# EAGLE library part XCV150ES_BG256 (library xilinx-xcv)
xcv150es_bg256 edit this description Auto generated by make-symbol-device-package-bsdl.ulp Rev. 26 Source: xcv150es_bg256.bsd
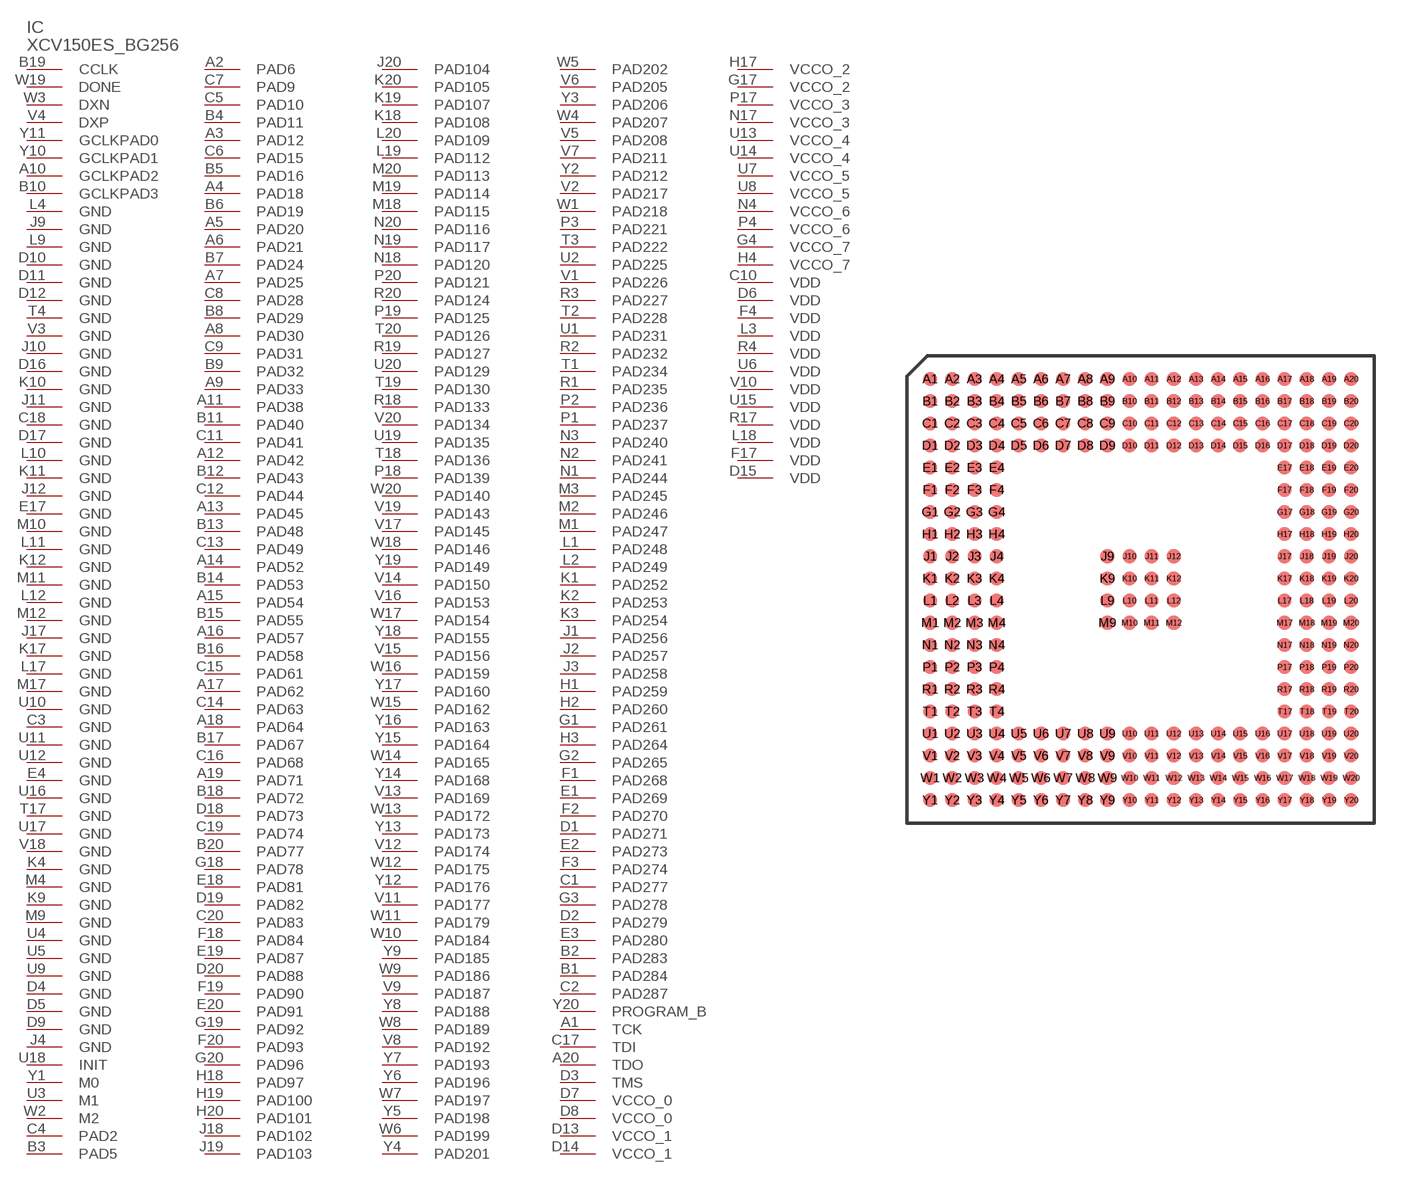
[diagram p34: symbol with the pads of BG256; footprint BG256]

Designator prefix IC

## XCV150ES_BG256 (OC_FARNELL: unknown; OC_NEWARK: unknown)  [BG256]
A1  TCK  in
A2  PAD6
A3  PAD12
A4  PAD18
A5  PAD20
A6  PAD21
A7  PAD25
A8  PAD30
A9  PAD33
A10  GCLKPAD2  in
A11  PAD38
A12  PAD42
A13  PAD45
A14  PAD52
A15  PAD54
A16  PAD57
A17  PAD62
A18  PAD64
A19  PAD71
A20  TDO  out
B1  PAD284
B2  PAD283
B3  PAD5
B4  PAD11
B5  PAD16
B6  PAD19
B7  PAD24
B8  PAD29
B9  PAD32
B10  GCLKPAD3  in
B11  PAD40
B12  PAD43
B13  PAD48
B14  PAD53
B15  PAD55
B16  PAD58
B17  PAD67
B18  PAD72
B19  CCLK
B20  PAD77
C1  PAD277
C2  PAD287
C3  GND  pwr
C4  PAD2
C5  PAD10
C6  PAD15
C7  PAD9
C8  PAD28
C9  PAD31
C10  VDD  pwr
C11  PAD41
C12  PAD44
C13  PAD49
C14  PAD63
C15  PAD61
C16  PAD68
C17  TDI  in
C18  GND  pwr
C19  PAD74
C20  PAD83
D1  PAD271
D2  PAD279
D3  TMS  in
D4  GND  pwr
D5  GND  pwr
D6  VDD  pwr
D7  VCCO_0  pwr
D8  VCCO_0  pwr
D9  GND  pwr
D10  GND  pwr
D11  GND  pwr
D12  GND  pwr
D13  VCCO_1  pwr
D14  VCCO_1  pwr
D15  VDD  pwr
D16  GND  pwr
D17  GND  pwr
D18  PAD73
D19  PAD82
D20  PAD88
E1  PAD269
E2  PAD273
E3  PAD280
E4  GND  pwr
E17  GND  pwr
E18  PAD81
E19  PAD87
E20  PAD91
F1  PAD268
F2  PAD270
F3  PAD274
F4  VDD  pwr
F17  VDD  pwr
F18  PAD84
F19  PAD90
F20  PAD93
G1  PAD261
G2  PAD265
G3  PAD278
G4  VCCO_7  pwr
G17  VCCO_2  pwr
G18  PAD78
G19  PAD92
G20  PAD96
H1  PAD259
H2  PAD260
H3  PAD264
H4  VCCO_7  pwr
H17  VCCO_2  pwr
H18  PAD97
H19  PAD100
H20  PAD101
J1  PAD256
J2  PAD257
J3  PAD258
J4  GND  pwr
J9  GND  pwr
J10  GND  pwr
J11  GND  pwr
J12  GND  pwr
J17  GND  pwr
J18  PAD102
J19  PAD103
J20  PAD104
K1  PAD252
K2  PAD253
K3  PAD254
K4  GND  pwr
K9  GND  pwr
K10  GND  pwr
K11  GND  pwr
K12  GND  pwr
K17  GND  pwr
K18  PAD108
K19  PAD107
K20  PAD105
L1  PAD248
L2  PAD249
L3  VDD  pwr
L4  GND  pwr
L9  GND  pwr
L10  GND  pwr
L11  GND  pwr
L12  GND  pwr
L17  GND  pwr
L18  VDD  pwr
L19  PAD112
L20  PAD109
M1  PAD247
M2  PAD246
M3  PAD245
M4  GND  pwr
M9  GND  pwr
M10  GND  pwr
M11  GND  pwr
M12  GND  pwr
M17  GND  pwr
M18  PAD115
M19  PAD114
M20  PAD113
N1  PAD244
N2  PAD241
N3  PAD240
N4  VCCO_6  pwr
N17  VCCO_3  pwr
N18  PAD120
N19  PAD117
N20  PAD116
P1  PAD237
P2  PAD236
P3  PAD221
P4  VCCO_6  pwr
P17  VCCO_3  pwr
P18  PAD139
P19  PAD125
P20  PAD121
R1  PAD235
R2  PAD232
R3  PAD227
R4  VDD  pwr
R17  VDD  pwr
R18  PAD133
R19  PAD127
R20  PAD124
T1  PAD234
T2  PAD228
T3  PAD222
T4  GND  pwr
T17  GND  pwr
T18  PAD136
T19  PAD130
T20  PAD126
U1  PAD231
U2  PAD225
U3  M1  in
U4  GND  pwr
U5  GND  pwr
U6  VDD  pwr
U7  VCCO_5  pwr
U8  VCCO_5  pwr
U9  GND  pwr
U10  GND  pwr
U11  GND  pwr
U12  GND  pwr
U13  VCCO_4  pwr
U14  VCCO_4  pwr
U15  VDD  pwr
U16  GND  pwr
U17  GND  pwr
U18  INIT
U19  PAD135
U20  PAD129
V1  PAD226
V2  PAD217
V3  GND  pwr
V4  DXP  pas
V5  PAD208
V6  PAD205
V7  PAD211
V8  PAD192
V9  PAD187
V10  VDD  pwr
V11  PAD177
V12  PAD174
V13  PAD169
V14  PAD150
V15  PAD156
V16  PAD153
V17  PAD145
V18  GND  pwr
V19  PAD143
V20  PAD134
W1  PAD218
W2  M2  in
W3  DXN  pas
W4  PAD207
W5  PAD202
W6  PAD199
W7  PAD197
W8  PAD189
W9  PAD186
W10  PAD184
W11  PAD179
W12  PAD175
W13  PAD172
W14  PAD165
W15  PAD162
W16  PAD159
W17  PAD154
W18  PAD146
W19  DONE
W20  PAD140
Y1  M0  in
Y2  PAD212
Y3  PAD206
Y4  PAD201
Y5  PAD198
Y6  PAD196
Y7  PAD193
Y8  PAD188
Y9  PAD185
Y10  GCLKPAD1  in
Y11  GCLKPAD0  in
Y12  PAD176
Y13  PAD173
Y14  PAD168
Y15  PAD164
Y16  PAD163
Y17  PAD160
Y18  PAD155
Y19  PAD149
Y20  PROGRAM_B  in

## Footprint BG256 (pad centres in mm)
xcv100_bg256_1532 edit this description Auto generated by make-symbol-device-package-bsdl.ulp Rev. 25 Source: xcv100_bg256_1532.bsd
smd 0.8 x 0.8: A1 -12.065,12.065; A2 -10.795,12.065; A3 -9.525,12.065; A4 -8.255,12.065; A5 -6.985,12.065; A6 -5.715,12.065; A7 -4.445,12.065; A8 -3.175,12.065; A9 -1.905,12.065; A10 -0.635,12.065; A11 0.635,12.065; A12 1.905,12.065; A13 3.175,12.065; A14 4.445,12.065; A15 5.715,12.065; A16 6.985,12.065; A17 8.255,12.065; A18 9.525,12.065; A19 10.795,12.065; A20 12.065,12.065; B1 -12.065,10.795; B2 -10.795,10.795; B3 -9.525,10.795; B4 -8.255,10.795; B5 -6.985,10.795; B6 -5.715,10.795; B7 -4.445,10.795; B8 -3.175,10.795; B9 -1.905,10.795; B10 -0.635,10.795; B11 0.635,10.795; B12 1.905,10.795; B13 3.175,10.795; B14 4.445,10.795; B15 5.715,10.795; B16 6.985,10.795; B17 8.255,10.795; B18 9.525,10.795; B19 10.795,10.795; B20 12.065,10.795; C1 -12.065,9.525; C2 -10.795,9.525; C3 -9.525,9.525; C4 -8.255,9.525; C5 -6.985,9.525; C6 -5.715,9.525; C7 -4.445,9.525; C8 -3.175,9.525; C9 -1.905,9.525; C10 -0.635,9.525; C11 0.635,9.525; C12 1.905,9.525; C13 3.175,9.525; C14 4.445,9.525; C15 5.715,9.525; C16 6.985,9.525; C17 8.255,9.525; C18 9.525,9.525; C19 10.795,9.525; C20 12.065,9.525; D1 -12.065,8.255; D2 -10.795,8.255; D3 -9.525,8.255; D4 -8.255,8.255; D5 -6.985,8.255; D6 -5.715,8.255; D7 -4.445,8.255; D8 -3.175,8.255; D9 -1.905,8.255; D10 -0.635,8.255; D11 0.635,8.255; D12 1.905,8.255; D13 3.175,8.255; D14 4.445,8.255; D15 5.715,8.255; D16 6.985,8.255; D17 8.255,8.255; D18 9.525,8.255; D19 10.795,8.255; D20 12.065,8.255; E1 -12.065,6.985; E2 -10.795,6.985; E3 -9.525,6.985; E4 -8.255,6.985; E17 8.255,6.985; E18 9.525,6.985; E19 10.795,6.985; E20 12.065,6.985; F1 -12.065,5.715; F2 -10.795,5.715; F3 -9.525,5.715; F4 -8.255,5.715; F17 8.255,5.715; F18 9.525,5.715; F19 10.795,5.715; F20 12.065,5.715; G1 -12.065,4.445; G2 -10.795,4.445; G3 -9.525,4.445; G4 -8.255,4.445; G17 8.255,4.445; G18 9.525,4.445; G19 10.795,4.445; G20 12.065,4.445; H1 -12.065,3.175; H2 -10.795,3.175; H3 -9.525,3.175; H4 -8.255,3.175; H17 8.255,3.175; H18 9.525,3.175; H19 10.795,3.175; H20 12.065,3.175; J1 -12.065,1.905; J2 -10.795,1.905; J3 -9.525,1.905; J4 -8.255,1.905; J9 -1.905,1.905; J10 -0.635,1.905; J11 0.635,1.905; J12 1.905,1.905; J17 8.255,1.905; J18 9.525,1.905; J19 10.795,1.905; J20 12.065,1.905; K1 -12.065,0.635; K2 -10.795,0.635; K3 -9.525,0.635; K4 -8.255,0.635; K9 -1.905,0.635; K10 -0.635,0.635; K11 0.635,0.635; K12 1.905,0.635; K17 8.255,0.635; K18 9.525,0.635; K19 10.795,0.635; K20 12.065,0.635; L1 -12.065,-0.635; L2 -10.795,-0.635; L3 -9.525,-0.635; L4 -8.255,-0.635; L9 -1.905,-0.635; L10 -0.635,-0.635; L11 0.635,-0.635; L12 1.905,-0.635; L17 8.255,-0.635; L18 9.525,-0.635; L19 10.795,-0.635; L20 12.065,-0.635; M1 -12.065,-1.905; M2 -10.795,-1.905; M3 -9.525,-1.905; M4 -8.255,-1.905; M9 -1.905,-1.905; M10 -0.635,-1.905; M11 0.635,-1.905; M12 1.905,-1.905; M17 8.255,-1.905; M18 9.525,-1.905; M19 10.795,-1.905; M20 12.065,-1.905; N1 -12.065,-3.175; N2 -10.795,-3.175; N3 -9.525,-3.175; N4 -8.255,-3.175; N17 8.255,-3.175; N18 9.525,-3.175; N19 10.795,-3.175; N20 12.065,-3.175; P1 -12.065,-4.445; P2 -10.795,-4.445; P3 -9.525,-4.445; P4 -8.255,-4.445; P17 8.255,-4.445; P18 9.525,-4.445; P19 10.795,-4.445; P20 12.065,-4.445; R1 -12.065,-5.715; R2 -10.795,-5.715; R3 -9.525,-5.715; R4 -8.255,-5.715; R17 8.255,-5.715; R18 9.525,-5.715; R19 10.795,-5.715; R20 12.065,-5.715; T1 -12.065,-6.985; T2 -10.795,-6.985; T3 -9.525,-6.985; T4 -8.255,-6.985; T17 8.255,-6.985; T18 9.525,-6.985; T19 10.795,-6.985; T20 12.065,-6.985; U1 -12.065,-8.255; U2 -10.795,-8.255; U3 -9.525,-8.255; U4 -8.255,-8.255; U5 -6.985,-8.255; U6 -5.715,-8.255; U7 -4.445,-8.255; U8 -3.175,-8.255; U9 -1.905,-8.255; U10 -0.635,-8.255; U11 0.635,-8.255; U12 1.905,-8.255; U13 3.175,-8.255; U14 4.445,-8.255; U15 5.715,-8.255; U16 6.985,-8.255; U17 8.255,-8.255; U18 9.525,-8.255; U19 10.795,-8.255; U20 12.065,-8.255; V1 -12.065,-9.525; V2 -10.795,-9.525; V3 -9.525,-9.525; V4 -8.255,-9.525; V5 -6.985,-9.525; V6 -5.715,-9.525; V7 -4.445,-9.525; V8 -3.175,-9.525; V9 -1.905,-9.525; V10 -0.635,-9.525; V11 0.635,-9.525; V12 1.905,-9.525; V13 3.175,-9.525; V14 4.445,-9.525; V15 5.715,-9.525; V16 6.985,-9.525; V17 8.255,-9.525; V18 9.525,-9.525; V19 10.795,-9.525; V20 12.065,-9.525; W1 -12.065,-10.795; W2 -10.795,-10.795; W3 -9.525,-10.795; W4 -8.255,-10.795; W5 -6.985,-10.795; W6 -5.715,-10.795; W7 -4.445,-10.795; W8 -3.175,-10.795; W9 -1.905,-10.795; W10 -0.635,-10.795; W11 0.635,-10.795; W12 1.905,-10.795; W13 3.175,-10.795; W14 4.445,-10.795; W15 5.715,-10.795; W16 6.985,-10.795; W17 8.255,-10.795; W18 9.525,-10.795; W19 10.795,-10.795; W20 12.065,-10.795; Y1 -12.065,-12.065; Y2 -10.795,-12.065; Y3 -9.525,-12.065; Y4 -8.255,-12.065; Y5 -6.985,-12.065; Y6 -5.715,-12.065; Y7 -4.445,-12.065; Y8 -3.175,-12.065; Y9 -1.905,-12.065; Y10 -0.635,-12.065; Y11 0.635,-12.065; Y12 1.905,-12.065; Y13 3.175,-12.065; Y14 4.445,-12.065; Y15 5.715,-12.065; Y16 6.985,-12.065; Y17 8.255,-12.065; Y18 9.525,-12.065; Y19 10.795,-12.065; Y20 12.065,-12.065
